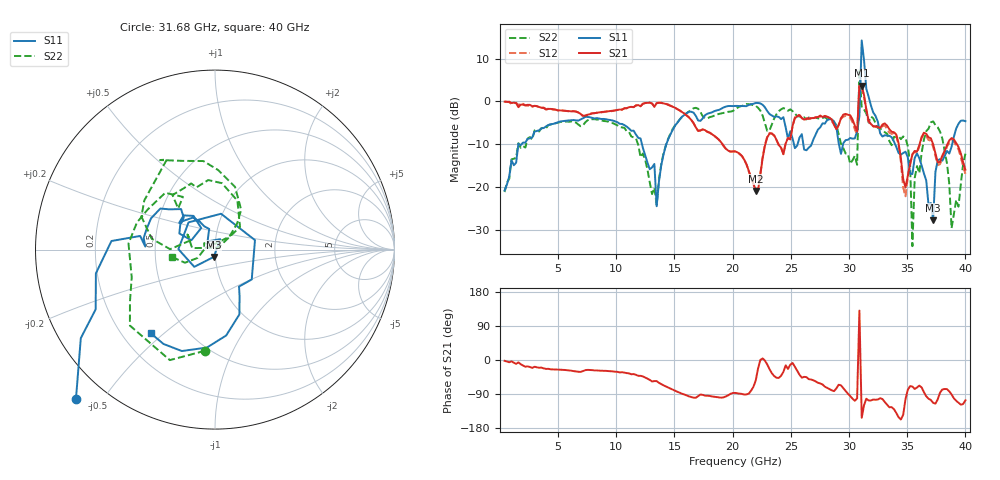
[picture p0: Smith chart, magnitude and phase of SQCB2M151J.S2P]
! Network Analyzer HP8722ES.07.66: Jul 25, 2000 Serial No. US39175408
! 27 Oct 2004  13:16:46
! Frequency  S11  S21  S12  S22
# HZ  S  DB R  50
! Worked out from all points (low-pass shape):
!   201 points, 400 MHz to 40 GHz, reference 50 ohm
!   highest |S21| = 3.71 dB at 31.09 GHz (marker M1); lowest = -21.0 dB at 21.98 GHz (marker M2)
!   |S21| within 3 dB of the highest: 30.84 GHz to 31.34 GHz (496.8 MHz wide, 1.6 % of centre)
!   lowest |S11| = -27.8 dB at 37.23 GHz (marker M3), VSWR 1.09, Z = 49.2 - j3.99 ohm
!   |S11| at or under -10 dB: start of sweep to 1.583 GHz; 12.2 GHz to 14.3 GHz (2.096 GHz wide, 15.8 % of centre); 33.96 GHz to 38.86 GHz (4.903 GHz wide, 13.5 % of centre)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
!   |S22| runs from -33.9 to 7.6 dB; largest |S21 - S12| = 0.26
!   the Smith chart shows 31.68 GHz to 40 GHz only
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4e8  -20.82 -96.9  -0.05 -2.3  -0.01 -1.7  -21.20 -93.2
7.132e9  -3.94 -105.0  -3.33 -29.3  -3.42 -30.2  -5.64 -115.6
1.3666e10  -18.71 -2.1  -0.32 -60.3  -0.26 -60.4  -18.22 35.4
1.5646e10  -3.57 1.7  -2.49 -89.1  -2.46 -89.2  -3.66 -6.3
2.02e10  -1.05 1.4  -11.66 -86.8  -11.72 -86.8  -1.91 -21.9
2.1982e10  -0.36 -5.9  -20.96 -54.0  -21.08 -51.7  -1.01 -38.0
2.4952e10  -6.98 -68.8  -8.90 -12.2  -8.80 -11.8  -1.84 -29.4
2.6932e10  -8.91 88.3  -3.91 -53.5  -3.98 -57.7  -3.90 -31.7
3.0694e10  -7.05 62.0  -6.99 -101.4  -7.74 -102.4  -14.82 -118.8
3.0892e10  -3.45 2.3  3.50 130.4  3.91 139.8  7.64 10.6
3.109e10  14.27 -95.0  3.71 -152.4  3.01 -152.2  -1.50 172.0
3.1288e10  9.67 -109.1  1.53 -119.3  1.09 -119.5  -1.87 -126.9
3.1486e10  2.97 -106.0  -1.83 -102.2  -2.18 -103.2  -2.81 -91.9
3.1684e10  1.10 -133.0  -4.52 -106.9  -4.79 -108.4  -4.93 -95.7
3.3466e10  -8.03 153.9  -6.50 -124.7  -7.30 -126.9  -9.28 121.3
3.505e10  -13.05 122.5  -17.43 -78.7  -17.65 -69.7  -10.46 65.4
3.5446e10  -16.98 158.5  -12.40 -70.0  -12.37 -69.1  -33.86 30.6
3.5644e10  -13.22 155.7  -11.57 -76.4  -11.74 -77.8  -17.90 176.2
3.7228e10  -27.77 -98.4  -10.00 -113.1  -10.62 -112.3  -4.65 121.5
3.7624e10  -13.80 179.3  -14.27 -103.6  -14.88 -102.3  -6.06 97.5
3.8812e10  -10.61 -62.3  -8.56 -90.9  -9.01 -90.4  -29.67 84.0
4e10  -4.62 -127.6  -15.96 -106.4  -16.91 -98.5  -12.23 -170.5
